(* Logix 5000 AddOnInstructionDefinition export Banner_K50Display_PD_v4; software revision 33.00 *)

TYPE Banner_K50Display_Advanced_PD_V4 :   // K50 Pro Display Advanced
STRUCT
   PDI_Output_Area_1 : SINT;   // 0 = Inactive,1 = Active
   PDI_Output_Area_2 : SINT;   // 0 = Inactive,1 = Active
   PDO_Animation : SINT;   // 0 = Off, 1 = Steady, 2 = Flash, 3 = 2 Color Flash, 4 = 50/50, 5 = 50/50 Rotate, 6 = Chase, 7 = Intensity Sweep, 8 = Color Sweep, 9 Sequence, 10 = Wave, 11 = Double Wave, 12 = Steady Area 1, 13 = Steady Area 2, 14 = Alternate Area1 Area 2
   PDO_Direction : SINT;   // 0 = CCW, 1 = CW
   PDO_Pattern : SINT;   // 0 = Flash, 1 = Strobe, 2 = 3 Pulse, 3 = SOS, 4 = Random
   PDO_Speed : SINT;   // 0 = Slow, 1 = Medium, 2 = Fast, 3 = Custom
   PDO_Dyanamic_Sequence : SINT;   // 0 to 255
   PDO_Sequence_Start_Location : SINT;   // 0 = LED1, 1 = LED2, 2 = LED3, 3 = LED4, 4 = LED5, 5 = LED6, 6 = LED7, 7 = LED8
   PDO_Color_1 : SINT;   // 0 = Green, 1 = Red, 2 = Orange, 3 = Amber, 4 = Yellow, 5 = Lime Green, 6 = Spring Green, 7 = Cyan, 8 = Sky Blue, 9 = Blue, 10 = Violet, 11 = Magenta, 12 = Rose, 13 = White, 14 = Custom 1, 15 = Custom 2
   PDO_Color_1_Intensity : SINT;   // 0 = High, 1 = Medium, 2 = Low, 3 = Off, 4 = Custom
   PDO_Color_2 : SINT;   // 0 = Green, 1 = Red, 2 = Orange, 3 = Amber, 4 = Yellow, 5 = Lime Green, 6 = Spring Green, 7 = Cyan, 8 = Sky Blue, 9 = Blue, 10 = Violet, 11 = Magenta, 12 = Rose, 13 = White, 14 = Custom 1, 15 = Custom 2.
   PDO_Color_2_Intensity : SINT;   // 0 = High, 1 = Medium, 2 = Low, 3 = Off, 4 = Custom
   PDO_Number : INT;
   PDO_String : STRING;
END_STRUCT
END_TYPE

TYPE Banner_K50Display_Four_PD_v4 :   // K50 Pro Display Four State Full Logic
STRUCT
   PDI_State : SINT;   // 0 = State 1, 1 = State 2, 2 = State 3, 3 = State 4
   PDI_State_Area_1 : SINT;   // 0 = Inactive, 1 = Active
   PDI_State_Area_2 : SINT;   // 0 = Inactive, 1 = Active
   PDO_Job_Input : SINT;   // 0 = Off, 1 = On
   PDO_Number : INT;
   PDO_String : STRING;
END_STRUCT
END_TYPE

TYPE Banner_K50Display_LED_v4 :   // LED Control Process Data for a K50 Pro Display.
STRUCT
   PDI_State_Area_1 : SINT;   // 0 = Inactive, 1 = Active.
   PDI_State_Area_2 : SINT;   // 0 = Inactive, 1 = Active.
   LED_1_Color : SINT;   // 0 = Green, 1 = Red, 2 = Orange, 3 = Amber, 4 = Yellow, 5 = Lime Green, 6 = Spring Green, 7 = Cyan, 8 = Sky Blue, 9 = Blue, 10 = Violet, 11 = Magenta, 12 = Rose, 13 = White, 14 = Custom 1, 15 = Custom 2.
   LED_1_Intensity : SINT;   // 0 to 10 (0 to 100%).
   LED_2_Color : SINT;   // 0 = Green, 1 = Red, 2 = Orange, 3 = Amber, 4 = Yellow, 5 = Lime Green, 6 = Spring Green, 7 = Cyan, 8 = Sky Blue, 9 = Blue, 10 = Violet, 11 = Magenta, 12 = Rose, 13 = White, 14 = Custom 1, 15 = Custom 2.
   LED_2_Intensity : SINT;   // 0 to 10 (0 to 100%).
   LED_3_Color : SINT;   // 0 = Green, 1 = Red, 2 = Orange, 3 = Amber, 4 = Yellow, 5 = Lime Green, 6 = Spring Green, 7 = Cyan, 8 = Sky Blue, 9 = Blue, 10 = Violet, 11 = Magenta, 12 = Rose, 13 = White, 14 = Custom 1, 15 = Custom 2.
   LED_3_Intensity : SINT;   // 0 to 10 (0 to 100%).
   LED_4_Color : SINT;   // 0 = Green, 1 = Red, 2 = Orange, 3 = Amber, 4 = Yellow, 5 = Lime Green, 6 = Spring Green, 7 = Cyan, 8 = Sky Blue, 9 = Blue, 10 = Violet, 11 = Magenta, 12 = Rose, 13 = White, 14 = Custom 1, 15 = Custom 2.
   LED_4_Intensity : SINT;   // 0 to 10 (0 to 100%).
   LED_5_Color : SINT;   // 0 = Green, 1 = Red, 2 = Orange, 3 = Amber, 4 = Yellow, 5 = Lime Green, 6 = Spring Green, 7 = Cyan, 8 = Sky Blue, 9 = Blue, 10 = Violet, 11 = Magenta, 12 = Rose, 13 = White, 14 = Custom 1, 15 = Custom 2.
   LED_5_Intensity : SINT;   // 0 to 10 (0 to 100%).
   LED_6_Color : SINT;   // 0 = Green, 1 = Red, 2 = Orange, 3 = Amber, 4 = Yellow, 5 = Lime Green, 6 = Spring Green, 7 = Cyan, 8 = Sky Blue, 9 = Blue, 10 = Violet, 11 = Magenta, 12 = Rose, 13 = White, 14 = Custom 1, 15 = Custom 2.
   LED_6_Intensity : SINT;   // 0 to 10 (0 to 100%).
   LED_7_Color : SINT;   // 0 = Green, 1 = Red, 2 = Orange, 3 = Amber, 4 = Yellow, 5 = Lime Green, 6 = Spring Green, 7 = Cyan, 8 = Sky Blue, 9 = Blue, 10 = Violet, 11 = Magenta, 12 = Rose, 13 = White, 14 = Custom 1, 15 = Custom 2.
   LED_7_Intensity : SINT;   // 0 to 10 (0 to 100%).
   LED_8_Color : SINT;   // 0 = Green, 1 = Red, 2 = Orange, 3 = Amber, 4 = Yellow, 5 = Lime Green, 6 = Spring Green, 7 = Cyan, 8 = Sky Blue, 9 = Blue, 10 = Violet, 11 = Magenta, 12 = Rose, 13 = White, 14 = Custom 1, 15 = Custom 2.
   LED_8_Intensity : SINT;   // 0 to 10 (0 to 100%).
   PDO_Number : INT;
   PDO_String : STRING;
END_STRUCT
END_TYPE

TYPE Banner_K50Display_Multi_PD_v4 :   // K50 Pro Display Multicolor Process Data
STRUCT
   PDI_State : SINT;   // 0 = State 1, 1 = State 2, 2 = State 3, 3 = State 4
   PDI_State_Area_1 : SINT;   // 0 = Inactive, 1 = Active
   PDI_State_Area_2 : SINT;   // 0 = Inactive, 1 = Active
   PDO_State : SINT;   // 0 = State 1, 1 = State 2, 2 = State 3, 3 = State 4
   PDO_Number : INT;
   PDO_String : STRING;
END_STRUCT
END_TYPE

TYPE Banner_K50Display_PDIO_v4 :   // UDT that records the converted prcoess data.
STRUCT
   PD_MultiColor : Banner_K50Display_Multi_PD_v4;   // Only active when Operation Mode set to 0. State tells the light which of the four states it should be in. 0 = State 1, 1 = State 2, 2 = State 3, 3 = State 4.
   PD_FourState : Banner_K50Display_Four_PD_v4;   // Only active when Operation Mode set to 1. Job Input tells the light how it should behave. 0 - Off, 1 = ON
   PD_Advanced : Banner_K50Display_Advanced_PD_V4;   // Only active when Operation Mode set to 2.
   PD_LED : Banner_K50Display_LED_v4;   // Only active when Operation Mode set to 3.
   PDO_DT : SINT[20];
   PDI_DT : SINT[2];
END_STRUCT
END_TYPE

ADD_ON_INSTRUCTION Banner_K50Display_PD_v4   (* revision 4.0, vendor Banner Engineering *)
// Takes the raw SINT information and converts that data into actual information.
VAR_IN_OUT
   PDIO : Banner_K50Display_PDIO_v4; {required}
END_VAR
VAR_INPUT
   Operation_Mode : SINT; {required}   // Linked from Parameters AOI or entered manually.
   Byte_Swap : BOOL; {required}
END_VAR
VAR
   PDO_Temp : SINT[20]; {access None}
   PDI_Temp : SINT[2]; {access None}
END_VAR

ROUTINE Logic   (* ladder *)
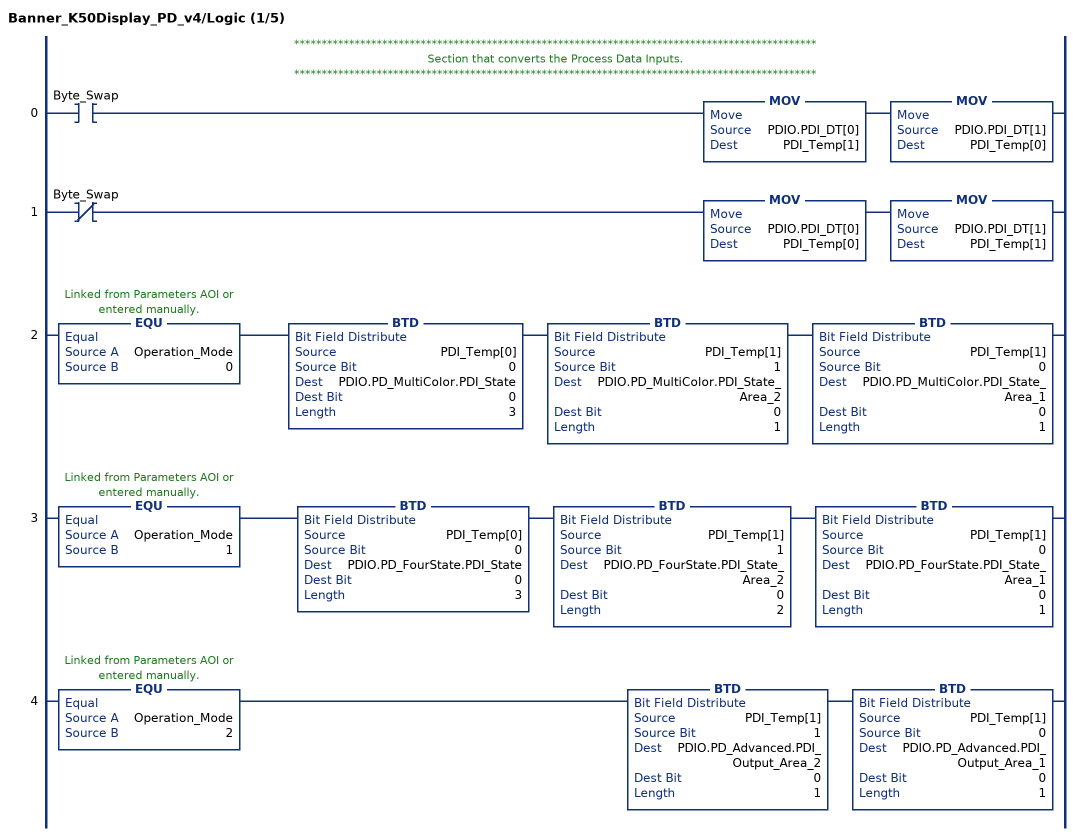
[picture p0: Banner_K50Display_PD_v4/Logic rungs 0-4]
   // ***********************************************************************************************
   // Section that converts the Process Data Inputs.
   // ***********************************************************************************************
   0: XIC(Byte_Swap)MOV(PDIO.PDI_DT[0],PDI_Temp[1])MOV(PDIO.PDI_DT[1],PDI_Temp[0]);
   1: XIO(Byte_Swap)MOV(PDIO.PDI_DT[0],PDI_Temp[0])MOV(PDIO.PDI_DT[1],PDI_Temp[1]);
   2: EQU(Operation_Mode,0)BTD(PDI_Temp[0],0,PDIO.PD_MultiColor.PDI_State,0,3)BTD(PDI_Temp[1],1,PDIO.PD_MultiColor.PDI_State_Area_2,0,1)BTD(PDI_Temp[1],0,PDIO.PD_MultiColor.PDI_State_Area_1,0,1);
   3: EQU(Operation_Mode,1)BTD(PDI_Temp[0],0,PDIO.PD_FourState.PDI_State,0,3)BTD(PDI_Temp[1],1,PDIO.PD_FourState.PDI_State_Area_2,0,2)BTD(PDI_Temp[1],0,PDIO.PD_FourState.PDI_State_Area_1,0,1);
   4: EQU(Operation_Mode,2)BTD(PDI_Temp[1],1,PDIO.PD_Advanced.PDI_Output_Area_2,0,1)BTD(PDI_Temp[1],0,PDIO.PD_Advanced.PDI_Output_Area_1,0,1);
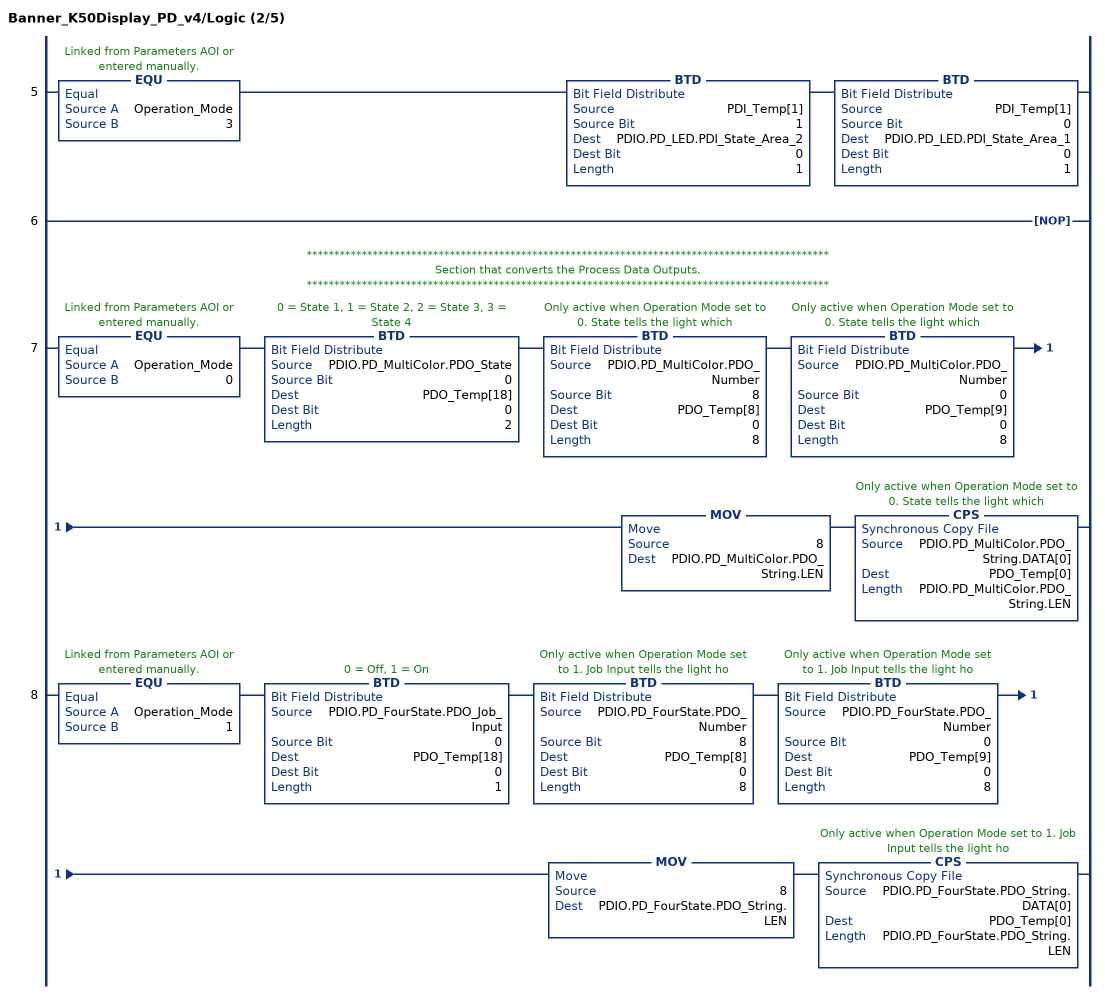
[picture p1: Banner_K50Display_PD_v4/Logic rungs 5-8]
   5: EQU(Operation_Mode,3)BTD(PDI_Temp[1],1,PDIO.PD_LED.PDI_State_Area_2,0,1)BTD(PDI_Temp[1],0,PDIO.PD_LED.PDI_State_Area_1,0,1);
   6: NOP();
   // ***********************************************************************************************
   // Section that converts the Process Data Outputs.
   // ***********************************************************************************************
   7: EQU(Operation_Mode,0)BTD(PDIO.PD_MultiColor.PDO_State,0,PDO_Temp[18],0,2)BTD(PDIO.PD_MultiColor.PDO_Number,8,PDO_Temp[8],0,8)BTD(PDIO.PD_MultiColor.PDO_Number,0,PDO_Temp[9],0,8)MOV(8,PDIO.PD_MultiColor.PDO_String.LEN)CPS(PDIO.PD_MultiColor.PDO_String.DATA[0],PDO_Temp[0],PDIO.PD_MultiColor.PDO_String.LEN);
   8: EQU(Operation_Mode,1)BTD(PDIO.PD_FourState.PDO_Job_Input,0,PDO_Temp[18],0,1)BTD(PDIO.PD_FourState.PDO_Number,8,PDO_Temp[8],0,8)BTD(PDIO.PD_FourState.PDO_Number,0,PDO_Temp[9],0,8)MOV(8,PDIO.PD_FourState.PDO_String.LEN)CPS(PDIO.PD_FourState.PDO_String.DATA[0],PDO_Temp[0],PDIO.PD_FourState.PDO_String.LEN);
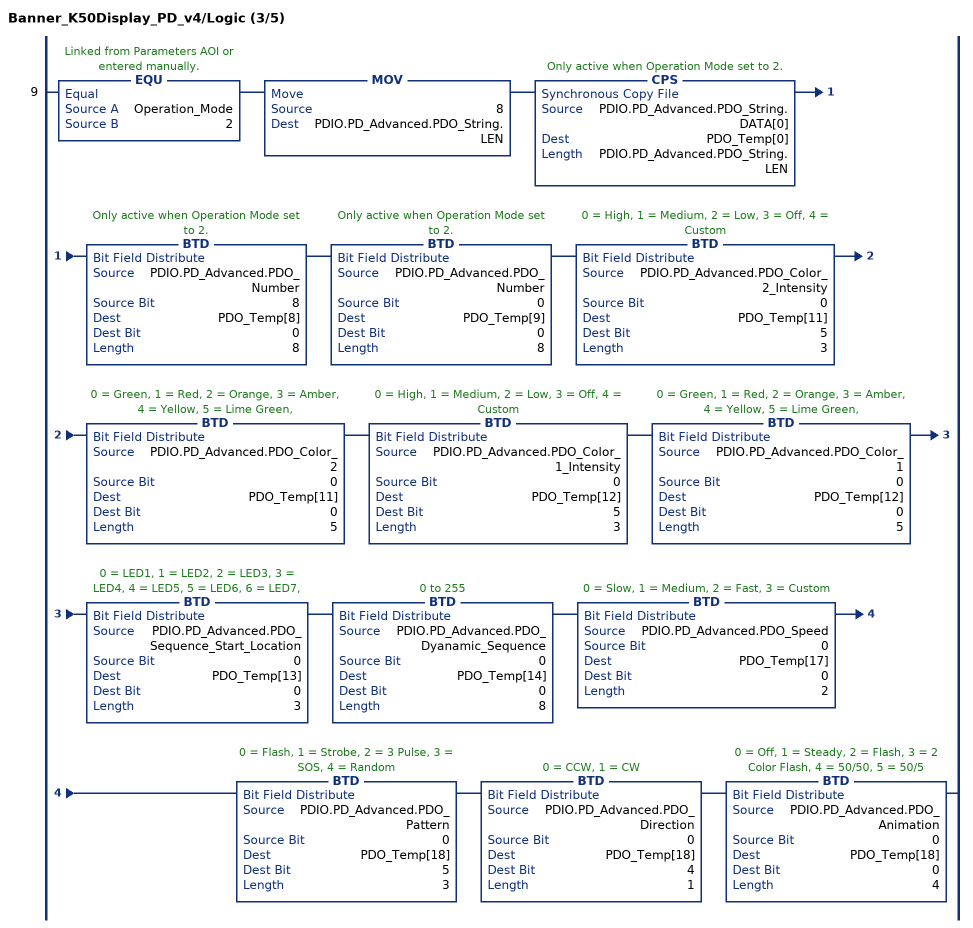
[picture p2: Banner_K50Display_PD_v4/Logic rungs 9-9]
   9: EQU(Operation_Mode,2)MOV(8,PDIO.PD_Advanced.PDO_String.LEN)CPS(PDIO.PD_Advanced.PDO_String.DATA[0],PDO_Temp[0],PDIO.PD_Advanced.PDO_String.LEN)BTD(PDIO.PD_Advanced.PDO_Number,8,PDO_Temp[8],0,8)BTD(PDIO.PD_Advanced.PDO_Number,0,PDO_Temp[9],0,8)BTD(PDIO.PD_Advanced.PDO_Color_2_Intensity,0,PDO_Temp[11],5,3)BTD(PDIO.PD_Advanced.PDO_Color_2,0,PDO_Temp[11],0,5)BTD(PDIO.PD_Advanced.PDO_Color_1_Intensity,0,PDO_Temp[12],5,3)BTD(PDIO.PD_Advanced.PDO_Color_1,0,PDO_Temp[12],0,5)BTD(PDIO.PD_Advanced.PDO_Sequence_Start_Location,0,PDO_Temp[13],0,3)BTD(PDIO.PD_Advanced.PDO_Dyanamic_Sequence,0,PDO_Temp[14],0,8)BTD(PDIO.PD_Advanced.PDO_Speed,0,PDO_Temp[17],0,2)BTD(PDIO.PD_Advanced.PDO_Pattern,0,PDO_Temp[18],5,3)BTD(PDIO.PD_Advanced.PDO_Direction,0,PDO_Temp[18],4,1)BTD(PDIO.PD_Advanced.PDO_Animation,0,PDO_Temp[18],0,4);
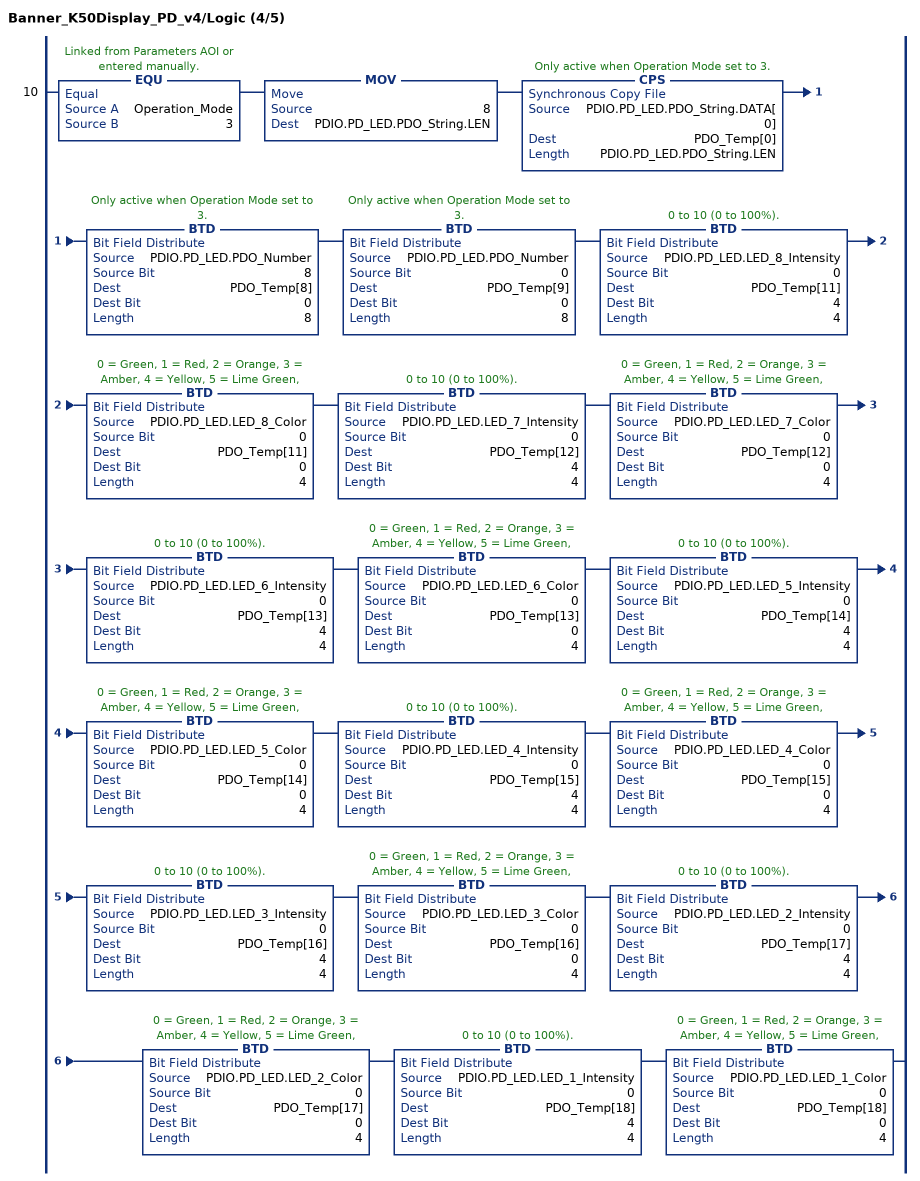
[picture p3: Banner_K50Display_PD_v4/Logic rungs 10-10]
   10: EQU(Operation_Mode,3)MOV(8,PDIO.PD_LED.PDO_String.LEN)CPS(PDIO.PD_LED.PDO_String.DATA[0],PDO_Temp[0],PDIO.PD_LED.PDO_String.LEN)BTD(PDIO.PD_LED.PDO_Number,8,PDO_Temp[8],0,8)BTD(PDIO.PD_LED.PDO_Number,0,PDO_Temp[9],0,8)BTD(PDIO.PD_LED.LED_8_Intensity,0,PDO_Temp[11],4,4)BTD(PDIO.PD_LED.LED_8_Color,0,PDO_Temp[11],0,4)BTD(PDIO.PD_LED.LED_7_Intensity,0,PDO_Temp[12],4,4)BTD(PDIO.PD_LED.LED_7_Color,0,PDO_Temp[12],0,4)BTD(PDIO.PD_LED.LED_6_Intensity,0,PDO_Temp[13],4,4)BTD(PDIO.PD_LED.LED_6_Color,0,PDO_Temp[13],0,4)BTD(PDIO.PD_LED.LED_5_Intensity,0,PDO_Temp[14],4,4)BTD(PDIO.PD_LED.LED_5_Color,0,PDO_Temp[14],0,4)BTD(PDIO.PD_LED.LED_4_Intensity,0,PDO_Temp[15],4,4)BTD(PDIO.PD_LED.LED_4_Color,0,PDO_Temp[15],0,4)BTD(PDIO.PD_LED.LED_3_Intensity,0,PDO_Temp[16],4,4)BTD(PDIO.PD_LED.LED_3_Color,0,PDO_Temp[16],0,4)BTD(PDIO.PD_LED.LED_2_Intensity,0,PDO_Temp[17],4,4)BTD(PDIO.PD_LED.LED_2_Color,0,PDO_Temp[17],0,4)BTD(PDIO.PD_LED.LED_1_Intensity,0,PDO_Temp[18],4,4)BTD(PDIO.PD_LED.LED_1_Color,0,PDO_Temp[18],0,4);
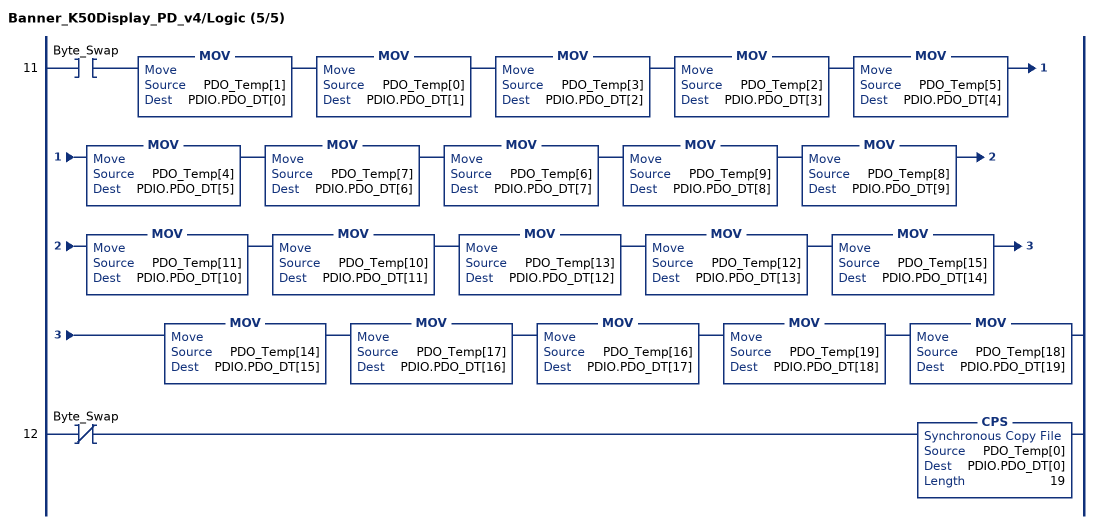
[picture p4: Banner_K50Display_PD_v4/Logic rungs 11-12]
   11: XIC(Byte_Swap)MOV(PDO_Temp[1],PDIO.PDO_DT[0])MOV(PDO_Temp[0],PDIO.PDO_DT[1])MOV(PDO_Temp[3],PDIO.PDO_DT[2])MOV(PDO_Temp[2],PDIO.PDO_DT[3])MOV(PDO_Temp[5],PDIO.PDO_DT[4])MOV(PDO_Temp[4],PDIO.PDO_DT[5])MOV(PDO_Temp[7],PDIO.PDO_DT[6])MOV(PDO_Temp[6],PDIO.PDO_DT[7])MOV(PDO_Temp[9],PDIO.PDO_DT[8])MOV(PDO_Temp[8],PDIO.PDO_DT[9])MOV(PDO_Temp[11],PDIO.PDO_DT[10])MOV(PDO_Temp[10],PDIO.PDO_DT[11])MOV(PDO_Temp[13],PDIO.PDO_DT[12])MOV(PDO_Temp[12],PDIO.PDO_DT[13])MOV(PDO_Temp[15],PDIO.PDO_DT[14])MOV(PDO_Temp[14],PDIO.PDO_DT[15])MOV(PDO_Temp[17],PDIO.PDO_DT[16])MOV(PDO_Temp[16],PDIO.PDO_DT[17])MOV(PDO_Temp[19],PDIO.PDO_DT[18])MOV(PDO_Temp[18],PDIO.PDO_DT[19]);
   12: XIO(Byte_Swap)CPS(PDO_Temp[0],PDIO.PDO_DT[0],19);
END_ROUTINE
END_ADD_ON_INSTRUCTION
